PROGRAM p06_frontDetection
VAR
	S0: BOOL;
	S1: BOOL;
	L0: BOOL;
	L1: BOOL;
	L2: BOOL;
	PositiveEdge: R_TRIG;
	NegativeEdge: F_TRIG;		
	PositiveFrontExpr: R_TRIG;
END_VAR

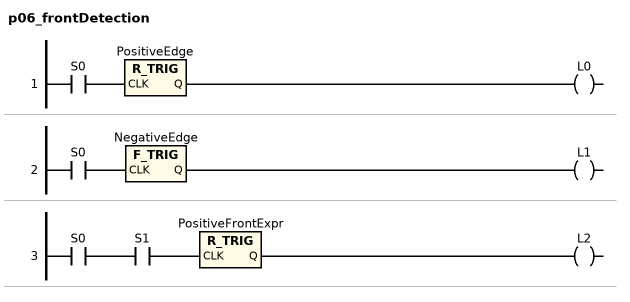
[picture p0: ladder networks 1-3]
// NETWORK 1
PositiveEdge(CLK := S0); // R_TRIG
L0 := PositiveEdge.Q;

// NETWORK 2
NegativeEdge(CLK := S0); // F_TRIG
L1 := NegativeEdge.Q;

// NETWORK 3
PositiveFrontExpr(CLK := S0 AND S1); // R_TRIG
L2 := PositiveFrontExpr.Q;

END_PROGRAM
